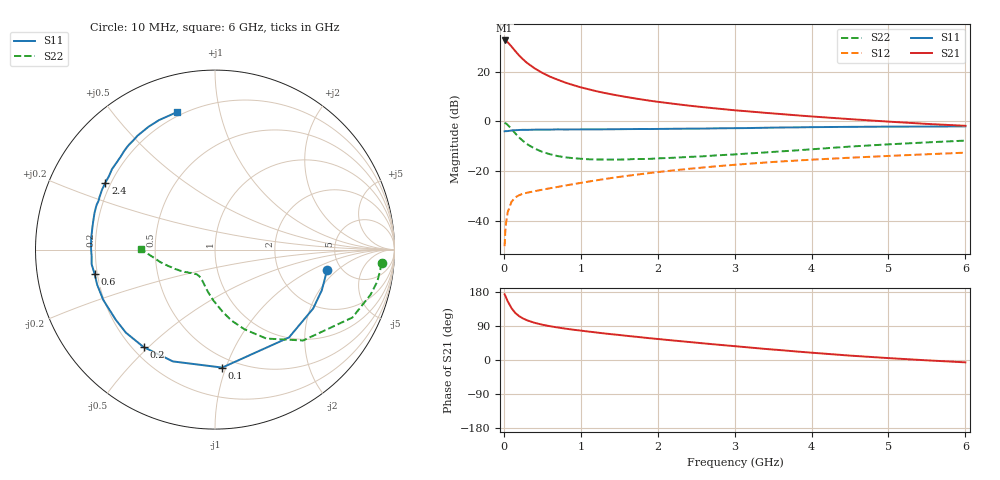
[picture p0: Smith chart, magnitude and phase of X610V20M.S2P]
! SIEMENS Small Signal Semiconductors
! BFP193W
! Si NPN RF Bipolar Junction Transistor in SOT343
! VCE = 10 V  IC = 20 mA
! Common Emitter S-Parameters:  April 1994
# GHz  S  MA  R  50
!  f  S11  S21  S12  S22
! GHz  MAG  ANG  MAG  ANG  MAG  ANG  MAG  ANG
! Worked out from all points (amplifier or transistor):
!   40 points, 10 MHz to 6 GHz, reference 50 ohm
!   highest |S21| = 32.6 dB at 10 MHz (marker M1)
!   |S21| within 3 dB of that: start of sweep to 115 MHz
!   unconditionally stable (mu >= 1): 1.054 GHz to 4.628 GHz
!   at 200 MHz: K = 0.34, MSG = 28.1 dB, |S12| = -29.7 dB
!   at 1.5 GHz: K = 1.09, MAG = 14.5 dB, |S12| = -22.3 dB
!   at 6 GHz: K = 0.95, MSG = 5.4 dB, |S12| = -12.6 dB
!   S11 on the Smith chart (normalised r, x): 10 MHz: 3.88, -1.48; 100 MHz: 0.42, -0.97; 200 MHz: 0.24, -0.48; 600 MHz: 0.19, -0.10; 2.4 GHz: 0.18, +0.27; 6 GHz: 0.18, +0.75
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0.01  0.635 -10.3  42.54 173.3  0.0031 75.8  0.9329 -4.6
0.02  0.6368 -20.8  42.11 169.2  0.0065 74.9  0.9219 -11.1
0.03  0.6378 -31.0  41.44 164.4  0.0093 74.4  0.9022 -16.2
0.05  0.6399 -49.9  39.12 155.0  0.0149 67.0  0.854 -26.3
0.1  0.6586 -86.5  32.14 136.7  0.0243 53.7  0.7052 -45.9
0.15  0.6656 -110.6  25.88 123.9  0.0298 45.6  0.5724 -60.0
0.2  0.6732 -126.2  21.1 115.5  0.0329 41.5  0.4734 -69.7
0.25  0.6787 -137.0  17.72 109.5  0.0353 38.8  0.405 -77.0
0.3  0.6772 -144.8  15.1 104.9  0.0368 38.2  0.351 -82.8
0.4  0.6829 -155.8  11.71 98.1  0.0396 37.7  0.2848 -91.6
0.5  0.685 -163.3  9.495 93.1  0.0424 39.7  0.2449 -98.3
0.6  0.6846 -168.7  7.966 89.2  0.0453 41.2  0.2189 -103.6
0.8  0.6885 -176.9  6.043 82.8  0.0515 44.5  0.1899 -111.1
1.1  0.6929 174.5  4.446 75.0  0.0617 48.3  0.1733 -119.5
1.3  0.6942 169.7  3.765 70.3  0.0691 50.0  0.1714 -123.1
1.6  0.7014 163.2  3.09 63.7  0.0804 51.2  0.172 -127.5
2.2  0.7124 152.1  2.272 51.5  0.1034 51.2  0.1858 -135.7
2.4  0.7158 148.6  2.084 47.7  0.1112 50.7  0.1932 -137.8
3.2  0.737 135.8  1.583 32.9  0.1417 47.1  0.2279 -149.0
4.5  0.7783 118.4  1.113 11.6  0.1864 39.6  0.3124 -167.1
5.5  0.7885 109.4  0.892 -0.9  0.2187 34.0  0.379 -176.9
6  0.7955 105.3  0.817 -6.2  0.2357 31.5  0.4117 179.3
